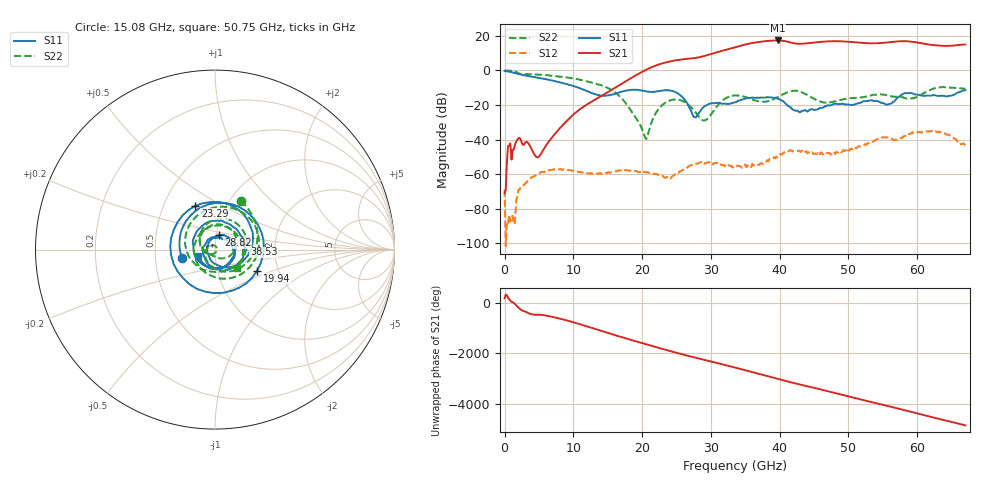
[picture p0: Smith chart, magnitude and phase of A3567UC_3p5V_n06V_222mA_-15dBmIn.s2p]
! MARKI MICROWAVE INC.
! Date:  4/20/2021
! Model Number:  A-3567UC
! Description:  2-port Small Signal S-parameter data for A-3567UC
! Frequency Range:  10 MHz to 67 GHz
! Port Configuration:  PORT 1: Input
!  PORT 2: Output
! Bias Condition: Vd = +3.5V, Vg = -0.6V, Id = 222mA
! A-3567UC s2p files are only valid for small signal conditions (below -10 dBm input power)
# Hz S  dB  R 50
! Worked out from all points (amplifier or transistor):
!   401 points, 10 MHz to 67 GHz, reference 50 ohm
!   highest |S21| = 17.3 dB at 39.7 GHz (marker M1)
!   |S21| within 3 dB of that: 34.34 GHz to 63.25 GHz (28.92 GHz wide, 59.3 % of centre)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
!   unconditionally stable (mu >= 1): 189.3 MHz to end of sweep
!   at 11.06 GHz: K = 3567.46, MAG = -20.3 dB, |S12| = -58.6 dB
!   at 33.51 GHz: K = 59.19, MAG = 13.7 dB, |S12| = -55.3 dB
!   at 67 GHz: K = 11.09, MAG = 15.6 dB, |S12| = -43.2 dB
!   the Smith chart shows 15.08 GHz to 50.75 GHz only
!   S11 on the Smith chart (normalised r, x): 15.08 GHz: 0.69, -0.07; 19.94 GHz: 1.56, -0.39; 23.29 GHz: 0.72, +0.38; 28.82 GHz: 1.03, +0.17; 38.53 GHz: 1.39, +0.09; 50.75 GHz: 0.82, -0.06
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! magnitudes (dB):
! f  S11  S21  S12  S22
! 10 MHz  -0.4  -71.1  -69.0  0.0
! 679.9 MHz  -0.7  -43.5  -83.6  -0.1
! 1.852 GHz  -1.9  -40.1  -72.3  -1.2
! 4.867 GHz  -4.2  -50.3  -59.9  -2.4
! 11.23 GHz  -10.7  -21.7  -59.0  -5.6
! 15.08 GHz  -14.4  -12.4  -58.9  -10.2
! 19.94 GHz  -11.6  -0.9  -58.7  -33.4
! 20.78 GHz  -12.2  0.8  -58.9  -37.9
! 22.45 GHz  -11.9  3.5  -60.7  -22.0
! 23.29 GHz  -11.5  4.5  -62.1  -18.9
! 25.63 GHz  -14.6  6.3  -58.2  -17.3
! 27.64 GHz  -27.0  7.2  -53.9  -23.6
! 28.82 GHz  -21.6  8.1  -53.3  -28.8
! 33.51 GHz  -18.4  13.4  -55.3  -14.5
! 38.53 GHz  -15.6  17.1  -51.1  -17.5
! 39.7 GHz  -16.4  17.3  -50.0  -15.4
! 44.73 GHz  -22.3  16.0  -47.3  -15.8
! 50.75 GHz  -19.8  16.4  -45.2  -15.9
! 55.95 GHz  -19.4  16.3  -38.8  -14.8
! 58.29 GHz  -13.1  16.9  -37.8  -16.1
! 62.81 GHz  -14.6  14.5  -35.5  -10.0
! 67 GHz  -11.5  15.0  -43.2  -10.6
